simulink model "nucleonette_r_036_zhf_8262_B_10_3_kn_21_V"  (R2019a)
settings: Solver=VariableStepAuto  StartTime=0.0  StopTime=727544.216  FixedStep=0.2  RelTol=1e-6
libraries: simulink x6
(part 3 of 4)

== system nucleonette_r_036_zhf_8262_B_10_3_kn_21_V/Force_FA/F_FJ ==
  In1 : Inport
  Add{12,37,39,52} (4 alike) : Sum
  Add33 : Sum  Inputs=-+
  C_10 : Constant  Value=10
  C_100 : Constant  Value=-100
  C_10_11 : Constant  Value=1E-21
  Clock1 : Clock
  Constant10 : Constant  Value=0.86602
  Constant13 : Constant  Value=3
  Constant15 : Constant  Value=1.0E-3
  Constant19 : Constant  Value=2
  Constant21 : Constant  Value=1.5
  Constant24 : Constant  Value=3
  Math Function25 : Math  Operator=square
  Math Function28 : Math  Operator=square
  Math Function33 : Math  Operator=pow
  Math Function38 : Math  Operator=pow
  Math Function4 : Math  Operator=square
  Math Function45 : Math  Operator=pow
  Nfjx/Dfjx_3 : Scope
  Omega_w1 : Constant  Value=0.00003453723537
  Product25 : Product  Inputs=**/
  Product28 : Product  Inputs=*/
  Product31 : Product  Inputs=/**
  Product{32,53,57,59,61} (5 alike) : Product
  Product44 : Product  Inputs=**/
  Product51 : Product  Inputs=*/*
  Product58 : Product  Inputs=3
  Sqrt11 : Sqrt
  Sqrt13 : Sqrt
  Trigonometric Function10 : Trigonometry  Operator=cos
  ex : Constant  Value=1.602176565
  kFJx : Constant  Value=7.39283526
  mFAx : Constant  Value=999.755388642
  rx1 : Constant  Value=0.36373
  Out1 : Outport
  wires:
  Sqrt11/1 -> Product51/3, Math Function33/1  "Dfj"
  Constant13/1 -> Sqrt13/1, Product32/2
  Constant15/1 -> Math Function45/1
  Product25/1 -> Product32/1  "r*cos(wt)/2"
  Add33/1 -> Math Function25/1
  kFJx/1 -> Product31/3
  Product59/1 -> Add12/1  "3*z/2"
  Add12/1 -> Math Function28/1, Product61/2  "Zfj"
  Product32/1 -> Add33/2  "3r*cos(wt)/2"
  Product61/1 -> Product28/1
  Constant24/1 -> Math Function33/2, Math Function45/2
  Add52/1 -> Product28/2  "Dfj_B"
  C_10_11/1 -> Add39/1
  Add39/1 -> Product53/1  "kn_Dfj"
  Math Function25/1 -> Add37/2
  Math Function28/1 -> Add37/1
  Math Function4/1 -> Product31/2
  Clock1/1 -> Product57/1
  Product58/1 -> Add12/2  "r*cos(wt)*sqrt(3)/2"
  Sqrt13/1 -> Product44/2  "sqrt(3)"
  C_100/1 -> Product51/1
  Product57/1 -> Trigonometric Function10/1  "angle_wt"
  Product44/1 -> Add33/1  "z*sqrt(3)/2"
  Math Function45/1 -> Add52/1
  Math Function33/1 -> Add52/2
  ex/1 -> Math Function4/1
  Constant19/1 -> Product25/3, Product44/3  "2"
  Trigonometric Function10/1 -> Product58/2, Product25/1  "cos(wt)"
  Constant10/1 -> Product58/1  "sqrt(3)/2"
  Product53/1 -> Product61/1
  Product28/1 -> Out1/1, Nfjx/Dfjx_3/1  "nfjx/dfjx_3"
  Omega_w1/1 -> Product57/2
  Add37/1 -> Sqrt11/1
  C_10/1 -> Math Function38/1
  Math Function38/1 -> Add39/2  "10_exp(-100Dfj/r)"
  Product51/1 -> Math Function38/2
  rx1/1 -> Product51/2, Product58/3, Product25/2  "rx"
  mFAx/1 -> Product31/1  "mx"
  Product31/1 -> Product53/2
  In1/1 -> Product59/2, Product44/1
  Constant21/1 -> Product59/1

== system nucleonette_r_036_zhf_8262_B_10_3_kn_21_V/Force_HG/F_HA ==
  In1 : Inport
  In2 : Inport  Port=2
  Add10 : Sum  Inputs=--+
  Add11 : Sum  Inputs=+-+
  Add15 : Sum
  Add19 : Sum
  Add20 : Sum
  Add3 : Sum  Inputs=+++
  Add7 : Sum  Inputs=-+
  C_100 : Constant  Value=-100
  C_10_11_1 : Constant  Value=1E-21
  Clock : Clock
  Constant1 : Constant  Value=10
  Constant15 : Constant  Value=1.0E-3
  Constant16 : Constant  Value=0.86602
  Constant22 : Constant  Value=2
  Constant24 : Constant  Value=3
  Constant5 : Constant  Value=2
  Constant8 : Constant  Value=3
  Constant9 : Constant  Value=3
  Math Function{2,7,9,13} (4 alike) : Math  Operator=square
  Math Function18 : Math  Operator=pow
  Math Function45 : Math  Operator=pow
  Math Function8 : Math  Operator=pow
  Nhax/Dhax_3 : Scope
  Omega_w : Constant  Value=0.00003453723537
  Product{1,16,43,74} (4 alike) : Product  Inputs=**
  Product{5,11,19,30,39} (5 alike) : Product
  Product22 : Product  Inputs=*/
  Product24 : Product  Inputs=*/
  Product35 : Product  Inputs=/**
  Product36 : Product  Inputs=/*
  Product38 : Product  Inputs=***
  Product41 : Product  Inputs=**/
  Product72 : Product  Inputs=*/*
  Sqrt1 : Sqrt
  Sqrt7 : Sqrt
  Subtract7 : Sum
  Trigonometric Function1 : Trigonometry
  Trigonometric Function2 : Trigonometry  Operator=cos
  Trigonometric Function3 : Trigonometry
  Trigonometric Function6 : Trigonometry  Operator=cos
  ex_1 : Constant  Value=1.602176565
  keHAx : Constant  Value=66.535517341
  mHG0 : Constant  Value=707.811386658
  rx : Constant  Value=0.36373
  Out1 : Outport
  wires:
  Product16/1 -> Add19/2  "r*sin(3wt)"
  Omega_w/1 -> Product5/2
  Subtract7/1 -> Product22/2
  Add20/1 -> Add7/2  "z/2 + z0 - z3"
  Math Function8/1 -> Subtract7/1  "Dhax_3"
  Product22/1 -> Nhax/Dhax_3/1, Out1/1  "nhax/dhax_3"
  keHAx/1 -> Product35/3
  Product1/1 -> Add10/1  "(z0-z3)*sqrt(3)/2"
  Trigonometric Function6/1 -> Product38/1, Product43/2  "cos(wt)"
  Add11/1 -> Math Function7/1  "Zha"
  Product43/1 -> Add10/3  "r*cos(wt)"
  Product41/1 -> Add10/2, Product30/1  "r*cos(3wt)/2"
  Product11/1 -> Add19/1  "r*sin(wt)"
  Math Function13/1 -> Product35/2
  Math Function18/1 -> Add15/1  "10_exp(-100Dha/r)"
  Trigonometric Function2/1 -> Product41/1  "cos(3wt)"
  Math Function9/1 -> Add3/2  "Xha_2"
  Product36/1 -> Add20/2  "z/2"
  Product24/1 -> Add11/1, Product1/2  "(z0-z3)/2"
  Constant8/1 -> Sqrt7/1, Product19/2
  Product39/1 -> Product22/1  "Nha"
  ex_1/1 -> Math Function13/1
  Product74/1 -> Product39/1  "kn_Dha"
  Trigonometric Function1/1 -> Product16/2  "sin(3wt)"
  Add3/1 -> Sqrt1/1  "Dhax_2"
  Math Function7/1 -> Add3/3  "Zha_2"
  Constant22/1 -> Product36/1
  Product38/1 -> Add7/1  "r*cos(wt)*sqrt(3)/2"
  Math Function2/1 -> Add3/1
  rx/1 -> Product41/2, Product43/1, Product72/2, Product38/2, Product16/1, Product11/2  "rx"
  Clock/1 -> Product5/1
  Add10/1 -> Math Function9/1  "Xha"
  Product72/1 -> Math Function18/2
  Constant16/1 -> Product38/3  "sqrt(3)/2"
  Trigonometric Function3/1 -> Product11/1  "sin(wt)"
  Product19/1 -> Trigonometric Function2/1, Trigonometric Function1/1
  Constant5/1 -> Product41/3, Product24/2  "2"
  Product35/1 -> Product74/2
  C_10_11_1/1 -> Add15/2
  mHG0/1 -> Product35/1  "mx"
  Add15/1 -> Product74/1
  Sqrt1/1 -> Math Function8/1, Product72/1  "Dhax"
  Sqrt7/1 -> Product30/2, Product1/1  "sqrt(3)"
  Constant9/1 -> Math Function8/2
  Add19/1 -> Math Function2/1  "r*sin(3wt) + r*sin(wt)"
  Product30/1 -> Add11/2  "r*cos(3wt)*sqrt(3)/2"
  Product5/1 -> Trigonometric Function6/1, Trigonometric Function3/1, Product19/1  "ai+wt"
  In2/1 -> Product24/1, Add20/1  "z0 - Z3"
  In1/1 -> Add11/3, Product36/2  "z"
  Add7/1 -> Product39/2
  C_100/1 -> Product72/3
  Constant1/1 -> Math Function18/1
  Constant15/1 -> Math Function45/1
  Constant24/1 -> Math Function45/2
  Math Function45/1 -> Subtract7/2

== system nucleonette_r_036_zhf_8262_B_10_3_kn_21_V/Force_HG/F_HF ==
  In1 : Inport
  In2 : Inport  Port=2
  Add13 : Sum  Inputs=+++
  Add14 : Sum  Inputs=+-+
  Add16 : Sum
  Add20 : Sum
  Add5 : Sum  Inputs=+++
  Add6 : Sum
  Add9 : Sum  Inputs=+-
  C_100 : Constant  Value=-100
  C_10_11_1 : Constant  Value=1E-21
  Clock : Clock
  Constant : Constant  Value=10
  Constant15 : Constant  Value=1.0E-3
  Constant16 : Constant  Value=0.86602
  Constant22 : Constant  Value=2
  Constant24 : Constant  Value=3
  Constant5 : Constant  Value=2
  Constant8 : Constant  Value=3
  Constant9 : Constant  Value=3
  Math Function{10..11,13,15} (4 alike) : Math  Operator=square
  Math Function12 : Math  Operator=pow
  Math Function19 : Math  Operator=pow
  Math Function45 : Math  Operator=pow
  Nhfx/Dhfx_3 : Scope
  Omega_w : Constant  Value=0.00003453723537
  Product{1,16,42..43,73} (5 alike) : Product  Inputs=**
  Product{5,19,30,37} (4 alike) : Product
  Product24 : Product  Inputs=*/
  Product34 : Product  Inputs=*/
  Product35 : Product  Inputs=/**
  Product36 : Product  Inputs=/*
  Product38 : Product  Inputs=***
  Product41 : Product  Inputs=**/
  Product49 : Product  Inputs=**/
  Sqrt7 : Sqrt
  Sqrt8 : Sqrt
  Subtract8 : Sum
  Trigonometric Function1 : Trigonometry
  Trigonometric Function2 : Trigonometry  Operator=cos
  Trigonometric Function5 : Trigonometry
  Trigonometric Function6 : Trigonometry  Operator=cos
  ex_1 : Constant  Value=1.602176565
  keHFx : Constant  Value=66.535517341
  mHG0 : Constant  Value=707.811386658
  rx : Constant  Value=0.36373
  Out1 : Outport
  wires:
  Constant15/1 -> Math Function45/1
  Product16/1 -> Add9/1  "r*sin(3wt)"
  Omega_w/1 -> Product5/2
  Add20/1 -> Add6/2  "z/2 + z0 - z3"
  keHFx/1 -> Product35/3
  Sqrt8/1 -> Product49/1, Math Function12/1  "Dhfx"
  Product1/1 -> Add13/1  "(z0-z3)*sqrt(3)/2"
  Add9/1 -> Math Function10/1  "r*sin(3wt) - r*sin(wt)"
  Trigonometric Function6/1 -> Product38/1, Product43/2  "cos(wt)"
  Add5/1 -> Sqrt8/1  "Dhfx_2"
  Product43/1 -> Add13/2  "r*cos(wt)"
  Product41/1 -> Product30/1, Add13/3  "r*cos(3wt)/2"
  Math Function13/1 -> Product35/2
  Trigonometric Function2/1 -> Product41/1  "cos(3wt)"
  Product36/1 -> Add20/2  "z/2"
  Product24/1 -> Add14/1, Product1/2  "(z0-z3)/2"
  Constant8/1 -> Sqrt7/1, Product19/2
  Product34/1 -> Out1/1, Nhfx/Dhfx_3/1  "Nhfx/Dhfx_3"
  ex_1/1 -> Math Function13/1
  Product5/1 -> Trigonometric Function6/1, Product19/1, Trigonometric Function5/1  "ai+wt"
  Product42/1 -> Add9/2  "r*sin(wt)"
  Trigonometric Function1/1 -> Product16/2  "sin(3wt)"
  Product73/1 -> Product37/1  "kn_Dhf"
  Trigonometric Function5/1 -> Product42/1  "sin(wt)"
  Math Function11/1 -> Add5/2  "Xhf_2"
  Add13/1 -> Math Function11/1  "Xhf"
  Constant22/1 -> Product36/1
  Product38/1 -> Add6/1  "r*cos(wt)*sqrt(3)/2"
  Constant24/1 -> Math Function45/2
  rx/1 -> Product38/2, Product49/3, Product42/2, Product43/1, Product16/1, Product41/2  "rx"
  Add16/1 -> Product73/1
  Clock/1 -> Product5/1
  Product37/1 -> Product34/1  "Nhf"
  Constant16/1 -> Product38/3  "sqrt(3)/2"
  Product19/1 -> Trigonometric Function2/1, Trigonometric Function1/1
  Constant5/1 -> Product24/2, Product41/3  "2"
  In2/1 -> Add20/1, Product24/1  "z0 - z3"
  Product35/1 -> Product73/2
  C_10_11_1/1 -> Add16/2
  mHG0/1 -> Product35/1  "mx"
  Add6/1 -> Product37/2
  Add14/1 -> Math Function15/1  "Zhf"
  Product49/1 -> Math Function19/2
  Math Function19/1 -> Add16/1  "10_exp(-100Dhf/r)"
  Sqrt7/1 -> Product30/2, Product1/1  "sqrt(3)"
  Math Function15/1 -> Add5/3  "Zhf_2"
  Constant9/1 -> Math Function12/2
  Product30/1 -> Add14/2  "r*cos(3wt)*sqrt(3)/2"
  Math Function10/1 -> Add5/1  "Yhf_2"
  Math Function45/1 -> Subtract8/2
  Math Function12/1 -> Subtract8/1  "Dhfx_3"
  Subtract8/1 -> Product34/2
  In1/1 -> Add14/3, Product36/2
  C_100/1 -> Product49/2
  Constant/1 -> Math Function19/1

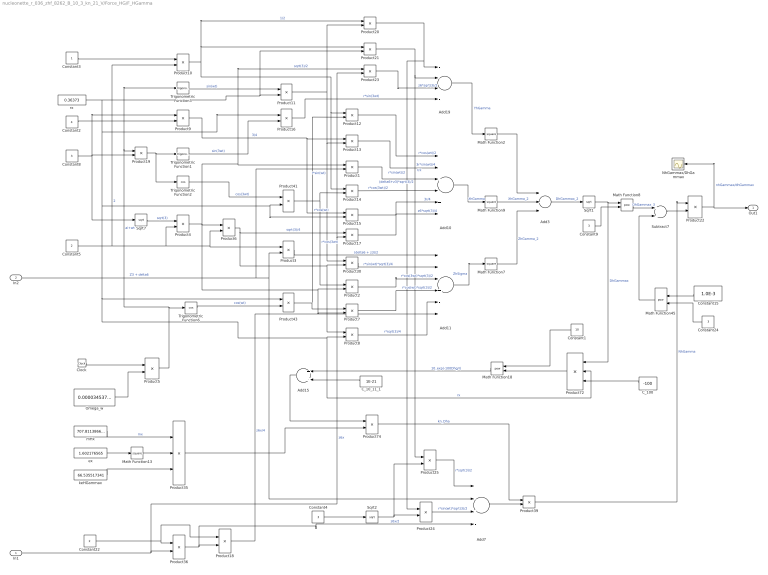
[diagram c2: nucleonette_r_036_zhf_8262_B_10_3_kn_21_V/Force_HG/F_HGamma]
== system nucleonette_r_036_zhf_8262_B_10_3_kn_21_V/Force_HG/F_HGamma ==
  In1 : Inport
  In2 : Inport  Port=2
  Add10 : Sum  Inputs=+-+-++
  Add11 : Sum  Inputs=-+-+--
  Add15 : Sum
  Add19 : Sum  Inputs=----
  Add3 : Sum  Inputs=+++
  Add7 : Sum  Inputs=--+-
  C_100 : Constant  Value=-100
  C_10_11_1 : Constant  Value=1E-21
  Clock : Clock
  Constant1 : Constant  Value=10
  Constant15 : Constant  Value=1.0E-3
  Constant2 : Constant  Value=4
  Constant22 : Constant  Value=2
  Constant{4,8..9,24} (4 alike) : Constant  Value=3
  Constant3 : Constant
  Constant5 : Constant  Value=2
  Math Function{2,7,9,13} (4 alike) : Math  Operator=square
  Math Function18 : Math  Operator=pow
  Math Function45 : Math  Operator=pow
  Math Function8 : Math  Operator=pow
  NhGammax/DhGammax : Scope
  Omega_w : Constant  Value=0.00003453723537
  Product{1,12..17,20..21,23..25,41,43,74} (15 alike) : Product  Inputs=**
  Product{4,6,9..10,22} (5 alike) : Product  Inputs=*/
  Product{2,5,7..8,11,19,30,39} (8 alike) : Product
  Product18 : Product  Inputs=/*
  Product3 : Product  Inputs=/*
  Product35 : Product  Inputs=/**
  Product36 : Product  Inputs=/*
  Product72 : Product  Inputs=*/*
  Sqrt1 : Sqrt
  Sqrt2 : Sqrt
  Sqrt7 : Sqrt
  Subtract7 : Sum
  Trigonometric Function1 : Trigonometry
  Trigonometric Function2 : Trigonometry  Operator=cos
  Trigonometric Function3 : Trigonometry
  Trigonometric Function6 : Trigonometry  Operator=cos
  ex : Constant  Value=1.602176565
  keHGammax : Constant  Value=66.535517341
  mHx : Constant  Value=707.811386658
  rx : Constant  Value=0.36373
  Out1 : Outport
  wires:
  Product15/1 -> Add10/5  "3r/4"
  Product18/1 -> Add11/6  "z6x/4"
  Constant4/1 -> Sqrt2/1
  Product4/1 -> Product7/2, Product2/2, Product6/1, Product23/1, Product1/1  "sqrt(3)/2"
  Product36/1 -> Add7/4, Product18/2  "z6x/2"
  Product3/1 -> Add11/1  "(delta6 + z3)/2"
  Constant2/1 -> Product9/2
  Product21/1 -> Add19/2, Product25/1  "r/2"
  Product23/1 -> Add19/3  "z6*sqrt(3)/2"
  Product16/1 -> Add19/4  "r*sin(3wt)"
  Product10/1 -> Product14/1, Product12/1, Product20/1, Product21/1  "1/2"
  Product13/1 -> Add10/2  "3r*sin(wt)/4"
  Product20/1 -> Add19/1, Product24/1  "r*sin(wt)/2"
  Sqrt2/1 -> Product25/2, Product24/2
  Product12/1 -> Add10/1  "r*cos(wt)/2"
  Product8/1 -> Add11/5  "r*sqrt(3)/4"
  Product7/1 -> Add11/4  "r*cos(wt)*sqrt(3)/2"
  Product9/1 -> Product15/1, Product13/1  "3/4"
  Product2/1 -> Add11/3  "r*cos(3wt)*sqrt(3)/2"
  Product6/1 -> Product17/1, Product8/1, Product30/2  "sqrt(3)/4"
  Product25/1 -> Add7/1  "r*sqrt(3)/2"
  Math Function45/1 -> Subtract7/2
  Constant24/1 -> Math Function45/2
  Constant1/1 -> Math Function18/1
  Constant15/1 -> Math Function45/1
  ex/1 -> Math Function13/1
  Add7/1 -> Product39/2
  C_10_11_1/1 -> Add15/2
  Add19/1 -> Math Function2/1  "YhGamma"
  Constant3/1 -> Product10/1
  Constant8/1 -> Product9/1, Sqrt7/1, Product19/2
  In1/1 -> Product17/2, Product23/2, Product36/2  "z6x"
  Product24/1 -> Add7/3  "r*sin(wt)*sqrt(3)/2"
  In2/1 -> Product1/2, Add7/2, Product3/2  "Z3 + delta6"
  Math Function7/1 -> Add3/3  "ZhGamma_2"
  Product19/1 -> Trigonometric Function2/1, Trigonometric Function1/1
  Subtract7/1 -> Product22/2
  Constant9/1 -> Math Function8/2
  Add15/1 -> Product74/1
  Product22/1 -> NhGammax/DhGammax/1, Out1/1  "nhGammax/dhGammax"
  Sqrt7/1 -> Product4/1  "sqrt(3)"
  Product35/1 -> Product74/2
  Product1/1 -> Add10/3  "(delta6+z3)*sqrt(3)/2"
  Constant5/1 -> Product10/2, Product4/2, Product3/1, Product6/2  "2"
  Trigonometric Function3/1 -> Product11/1  "sin(wt)"
  Product5/1 -> Trigonometric Function6/1, Trigonometric Function3/1, Product19/1  "ai+wt"
  Product30/1 -> Add11/2  "r*sin(wt)*sqrt(3)/4"
  Product43/1 -> Product12/2, Product7/1  "r*cos(wt)"
  Product41/1 -> Product14/2, Product2/1  "r*cos(3wt)"
  Product72/1 -> Math Function18/2
  Add10/1 -> Math Function9/1  "XhGamma"
  Clock/1 -> Product5/1
  rx/1 -> Product43/1, Product8/2, Product72/2, Product15/2, Product41/2, Product16/1, Product21/2, Product11/2  "rx"
  Trigonometric Function6/1 -> Product43/2  "cos(wt)"
  Math Function2/1 -> Add3/1
  Constant22/1 -> Product18/1, Product36/1
  Math Function18/1 -> Add15/1  "10_exp(-100Dhg/r)"
  Sqrt1/1 -> Math Function8/1, Product72/1  "DhGammax"
  Trigonometric Function1/1 -> Product16/2  "sin(3wt)"
  Add3/1 -> Sqrt1/1  "DhGammax_2"
  Product17/1 -> Add10/6  "z6*sqrt(3)/4"
  Product74/1 -> Product39/1  "kn_Dha"
  C_100/1 -> Product72/3
  Product39/1 -> Product22/1  "NhGamma"
  Add11/1 -> Math Function7/1  "ZhSigma"
  Trigonometric Function2/1 -> Product41/1  "cos(3wt)"
  Math Function9/1 -> Add3/2  "XhGamma_2"
  keHGammax/1 -> Product35/3
  Product11/1 -> Product13/2, Product30/1, Product20/2  "r*sin(wt)"
  Math Function8/1 -> Subtract7/1  "DhGammax_3"
  Math Function13/1 -> Product35/2
  Product14/1 -> Add10/4  "r*cos(3wt)/2"
  mHx/1 -> Product35/1  "mx"
  Omega_w/1 -> Product5/2

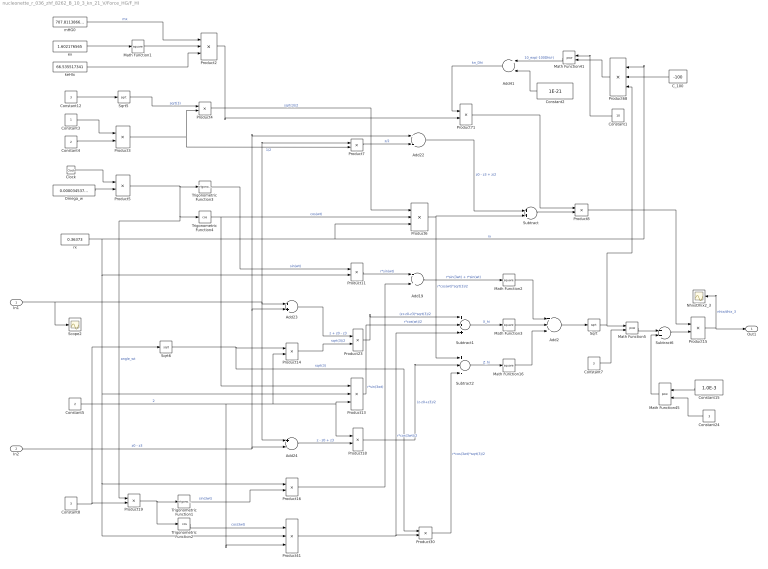
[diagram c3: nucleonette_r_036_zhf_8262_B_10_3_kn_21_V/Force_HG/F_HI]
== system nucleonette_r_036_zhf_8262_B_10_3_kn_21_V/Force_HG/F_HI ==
  In1 : Inport
  In2 : Inport  Port=2
  Add{19,22..23,41} (4 alike) : Sum
  Add2 : Sum  Inputs=+++
  Add24 : Sum  Inputs=+-
  C_100 : Constant  Value=-100
  Clock : Clock
  Constant1 : Constant  Value=10
  Constant{7..8,12,24} (4 alike) : Constant  Value=3
  Constant15 : Constant  Value=1.0E-3
  Constant2 : Constant  Value=1E-21
  Constant3 : Constant
  Constant4 : Constant  Value=2
  Constant5 : Constant  Value=2
  Math Function{1..3,16} (4 alike) : Math  Operator=square
  Math Function41 : Math  Operator=pow
  Math Function45 : Math  Operator=pow
  Math Function5 : Math  Operator=pow
  Nhix/Dhix2_3 : Scope
  Omega_w : Constant  Value=0.00003453723537
  Product{4..5,7..8,11,19,30,71} (8 alike) : Product
  Product13 : Product  Inputs=**/
  Product14 : Product  Inputs=*/
  Product15 : Product  Inputs=*/
  Product16 : Product  Inputs=**
  Product18 : Product  Inputs=/*
  Product2 : Product  Inputs=/**
  Product23 : Product  Inputs=**
  Product3 : Product  Inputs=*/
  Product41 : Product  Inputs=**/
  Product6 : Product  Inputs=3
  Product68 : Product  Inputs=/**
  Scope2 : Scope
  Sqrt : Sqrt
  Sqrt5 : Sqrt
  Sqrt6 : Sqrt
  Subtract : Sum
  Subtract1 : Sum  Inputs=+++
  Subtract2 : Sum  Inputs=+--
  Subtract6 : Sum
  Trigonometric Function1 : Trigonometry
  Trigonometric Function2 : Trigonometry  Operator=cos
  Trigonometric Function3 : Trigonometry
  Trigonometric Function4 : Trigonometry  Operator=cos
  ex : Constant  Value=1.602176565
  keHIx : Constant  Value=66.535517341
  mHG0 : Constant  Value=707.811386658
  rx : Constant  Value=0.36373
  Out1 : Outport
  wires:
  Sqrt5/1 -> Product4/1  "sqrt(3)"
  Product3/1 -> Product4/2, Product7/2  "1/2"
  Constant15/1 -> Math Function45/1
  Sqrt6/1 -> Product30/1, Product14/1  "sqrt(3)"
  Product41/1 -> Product30/2, Subtract1/3  "r*cos(3wt)/2"
  Subtract/1 -> Product8/2
  Subtract2/1 -> Math Function16/1  "Z_hi"
  Trigonometric Function3/1 -> Product11/1  "sin(wt)"
  Constant7/1 -> Math Function5/2
  Product8/1 -> Product15/1
  Constant24/1 -> Math Function45/2
  Constant4/1 -> Product3/2
  Product13/1 -> Subtract1/2  "r*cos(wt)/2"
  Product2/1 -> Product71/2
  Product6/1 -> Subtract/2, Subtract2/1  "r*cos(wt)*sqrt(3)/2"
  Add41/1 -> Product71/1  "kn_Dhi"
  Product11/1 -> Add19/1  "r*sin(wt)"
  Subtract6/1 -> Product15/2
  Add24/1 -> Product18/2  "z - z0 + z3"
  Math Function41/1 -> Add41/1  "10_exp(-100Dhi/r)"
  Product18/1 -> Subtract2/2  "(z-z0+z3)/2"
  Product14/1 -> Product23/2  "sqrt(3)/2"
  Constant8/1 -> Sqrt6/1, Product19/2
  Product71/1 -> Product8/1
  Add2/1 -> Sqrt/1
  Product4/1 -> Product6/1  "sqrt(3)/2"
  Product23/1 -> Subtract1/1  "(z+z0-z3)*sqrt(3)/2"
  mHG0/1 -> Product2/1  "mx"
  Add22/1 -> Subtract/1  "z0 - z3 + z/2"
  Add19/1 -> Math Function2/1  "r*sin(3wt) + r*sin(wt)"
  Subtract1/1 -> Math Function3/1  "X_hi"
  Omega_w/1 -> Product5/2
  Product19/1 -> Trigonometric Function2/1, Trigonometric Function1/1
  Add23/1 -> Product23/1  "z + z0 - z3"
  keHIx/1 -> Product2/3
  Sqrt/1 -> Math Function5/1, Product68/3
  ex/1 -> Math Function1/1
  Math Function45/1 -> Subtract6/2
  Math Function1/1 -> Product2/2
  Product68/1 -> Math Function41/2
  Math Function16/1 -> Add2/3
  Constant3/1 -> Product3/1
  Trigonometric Function1/1 -> Product16/2  "sin(3wt)"
  Math Function5/1 -> Subtract6/1
  Constant12/1 -> Sqrt5/1
  Product16/1 -> Add19/2  "r*sin(3wt)"
  rx/1 -> Product6/3, Product68/1, Product13/2, Product41/2, Product16/1, Product11/2  "rx"
  Math Function3/1 -> Add2/2
  Product5/1 -> Product19/1, Trigonometric Function4/1, Trigonometric Function3/1  "angle_wt"
  Product15/1 -> Out1/1, Nhix/Dhix2_3/1  "nhix/dhix_3"
  Product30/1 -> Subtract2/3  "r*cos(3wt)*sqrt(3)/2"
  Math Function2/1 -> Add2/1
  Product7/1 -> Add22/2  "z/2"
  Trigonometric Function4/1 -> Product13/1, Product6/2  "cos(wt)"
  C_100/1 -> Product68/2
  Constant5/1 -> Product41/3, Product14/2, Product18/1, Product13/3  "2"
  Clock/1 -> Product5/1
  Trigonometric Function2/1 -> Product41/1  "cos(3wt)"
  In1/1 -> Scope2/1, Product7/1, Add24/1, Add23/1
  In2/1 -> Add22/1, Add23/2, Add24/2  "z0 - z3"
  Constant1/1 -> Math Function41/1
  Constant2/1 -> Add41/2

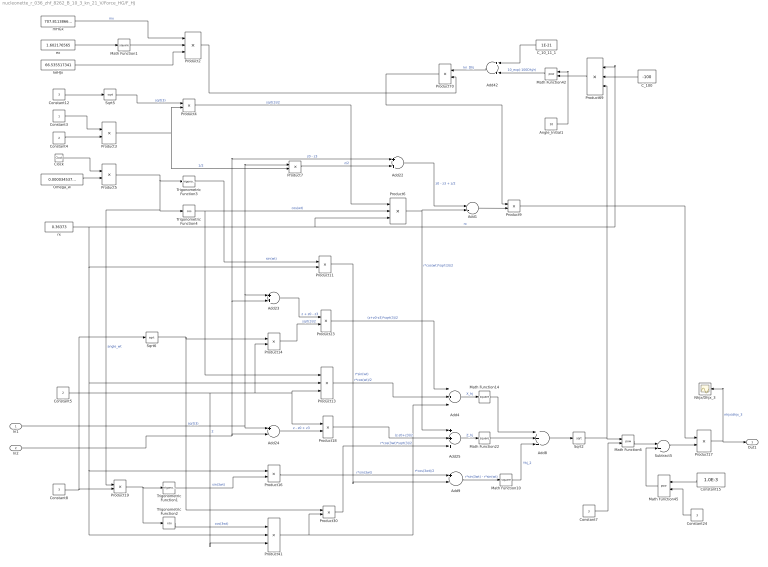
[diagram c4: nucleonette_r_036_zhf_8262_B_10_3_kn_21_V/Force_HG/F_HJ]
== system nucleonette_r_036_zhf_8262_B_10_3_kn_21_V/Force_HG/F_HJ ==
  In1 : Inport
  In2 : Inport  Port=2
  Add1 : Sum  Inputs=+-
  Add22 : Sum
  Add23 : Sum
  Add24 : Sum  Inputs=+-
  Add25 : Sum  Inputs=+++
  Add4 : Sum  Inputs=-+-
  Add42 : Sum
  Add8 : Sum  Inputs=+++
  Add9 : Sum  Inputs=+-
  Angle_Initial1 : Constant  Value=10
  C_100 : Constant  Value=-100
  C_10_11_1 : Constant  Value=1E-21
  Clock : Clock
  Constant{7..8,12,24} (4 alike) : Constant  Value=3
  Constant15 : Constant  Value=1.0E-3
  Constant3 : Constant
  Constant4 : Constant  Value=2
  Constant5 : Constant  Value=2
  Math Function{1,10,14,22} (4 alike) : Math  Operator=square
  Math Function42 : Math  Operator=pow
  Math Function45 : Math  Operator=pow
  Math Function6 : Math  Operator=pow
  Nhjx/Dhjx_3 : Scope
  Omega_w : Constant  Value=0.00003453723537
  Product{4..5,7,9,11,19,30,70} (8 alike) : Product
  Product13 : Product  Inputs=**/
  Product14 : Product  Inputs=*/
  Product16 : Product  Inputs=**
  Product17 : Product  Inputs=*/
  Product18 : Product  Inputs=/*
  Product2 : Product  Inputs=/**
  Product23 : Product  Inputs=**
  Product3 : Product  Inputs=*/
  Product41 : Product  Inputs=**/
  Product6 : Product  Inputs=3
  Product69 : Product  Inputs=/**
  Sqrt2 : Sqrt
  Sqrt5 : Sqrt
  Sqrt6 : Sqrt
  Subtract5 : Sum
  Trigonometric Function1 : Trigonometry
  Trigonometric Function2 : Trigonometry  Operator=cos
  Trigonometric Function3 : Trigonometry
  Trigonometric Function4 : Trigonometry  Operator=cos
  ex : Constant  Value=1.602176565
  keHJx : Constant  Value=66.535517341
  mHGx : Constant  Value=707.811386658
  rx : Constant  Value=0.36373
  Out1 : Outport
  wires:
  Product70/1 -> Product9/1
  Sqrt2/1 -> Product69/3, Math Function6/1
  Sqrt5/1 -> Product4/1  "sqrt(3)"
  Product3/1 -> Product4/2, Product7/2  "1/2"
  Constant15/1 -> Math Function45/1
  Sqrt6/1 -> Product14/1, Product30/1  "sqrt(3)"
  Product41/1 -> Product30/2, Add4/3  "r*cos(3wt)/2"
  Trigonometric Function3/1 -> Product11/1  "sin(wt)"
  Constant7/1 -> Math Function6/2
  Constant24/1 -> Math Function45/2
  Constant4/1 -> Product3/2
  Product13/1 -> Add4/2  "r*cos(wt)/2"
  Product2/1 -> Product70/2
  Product6/1 -> Add25/1, Add1/2  "r*cos(wt)*sqrt(3)/2"
  Product11/1 -> Add9/2  "r*sin(wt)"
  Add24/1 -> Product18/2  "z - z0 + z3"
  Product18/1 -> Add25/2  "(z-z0+z3)/2"
  Product14/1 -> Product23/2  "sqrt(3)/2"
  Math Function14/1 -> Add8/1
  Constant8/1 -> Sqrt6/1, Product19/2
  Add4/1 -> Math Function14/1  "X_hj"
  Product4/1 -> Product6/1  "sqrt(3)/2"
  Product23/1 -> Add4/1  "(z+z0-z3)*sqrt(3)/2"
  mHGx/1 -> Product2/1  "mx"
  Add22/1 -> Add1/1  "z0 - z3 + z/2"
  Product69/1 -> Math Function42/2
  Subtract5/1 -> Product17/2
  Omega_w/1 -> Product5/2
  Math Function22/1 -> Add8/2
  Product19/1 -> Trigonometric Function2/1, Trigonometric Function1/1
  Add23/1 -> Product23/1  "z + z0 - z3"
  Add42/1 -> Product70/1  "kn_Dhj"
  keHJx/1 -> Product2/3
  Add25/1 -> Math Function22/1  "Z_hj"
  Math Function42/1 -> Add42/2  "10_exp(-100Dhj/r)"
  ex/1 -> Math Function1/1
  Math Function45/1 -> Subtract5/2
  Math Function6/1 -> Subtract5/1
  Math Function1/1 -> Product2/2
  Product17/1 -> Out1/1, Nhjx/Dhjx_3/1  "nhjx/dhjx_3"
  Add8/1 -> Sqrt2/1
  Constant3/1 -> Product3/1
  Trigonometric Function1/1 -> Product16/2  "sin(3wt)"
  Constant12/1 -> Sqrt5/1
  Product16/1 -> Add9/1  "r*sin(3wt)"
  Add1/1 -> Product9/2
  rx/1 -> Product13/2, Product41/2, Product16/1, Product11/2, Product6/3, Product69/1  "rx"
  Add9/1 -> Math Function10/1  "r*sin(3wt) - r*sin(wt)"
  Product5/1 -> Trigonometric Function3/1, Trigonometric Function4/1, Product19/1  "angle_wt"
  Product30/1 -> Add25/3  "r*cos(3wt)*sqrt(3)/2"
  Product7/1 -> Add22/2  "z/2"
  Trigonometric Function4/1 -> Product13/1, Product6/2  "cos(wt)"
  C_100/1 -> Product69/2
  Product9/1 -> Product17/1
  Constant5/1 -> Product41/3, Product14/2, Product13/3, Product18/1  "2"
  Math Function10/1 -> Add8/3  "Yhj_2"
  Clock/1 -> Product5/1
  Trigonometric Function2/1 -> Product41/1  "cos(3wt)"
  C_10_11_1/1 -> Add42/1
  In1/1 -> Product7/1, Add23/1, Add24/1
  In2/1 -> Add22/1, Add23/2, Add24/2  "z0 - z3"
  Angle_Initial1/1 -> Math Function42/1

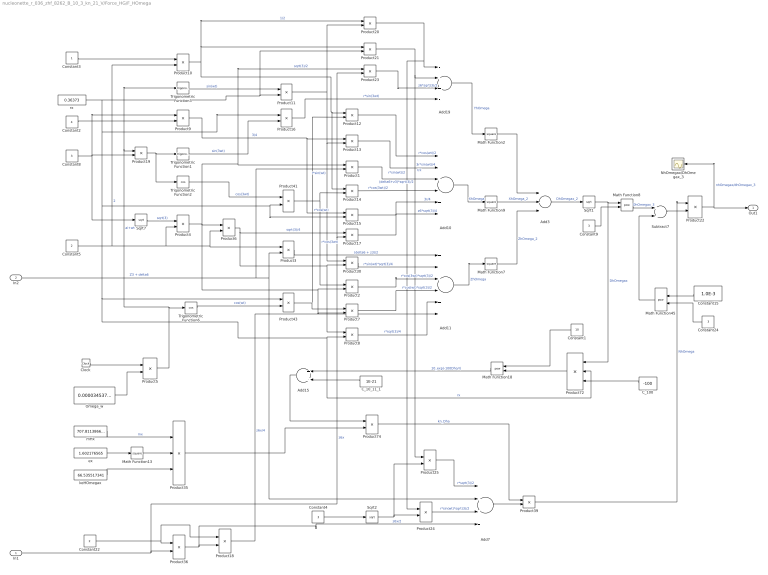
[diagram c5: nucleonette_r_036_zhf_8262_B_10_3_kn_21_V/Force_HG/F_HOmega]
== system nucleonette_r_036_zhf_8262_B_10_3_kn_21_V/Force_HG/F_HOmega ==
  In1 : Inport
  In2 : Inport  Port=2
  Add10 : Sum  Inputs=+++-++
  Add11 : Sum  Inputs=+++-++
  Add15 : Sum
  Add19 : Sum  Inputs=-++-
  Add3 : Sum  Inputs=+++
  Add7 : Sum  Inputs=++++
  C_100 : Constant  Value=-100
  C_10_11_1 : Constant  Value=1E-21
  Clock : Clock
  Constant1 : Constant  Value=10
  Constant15 : Constant  Value=1.0E-3
  Constant2 : Constant  Value=4
  Constant22 : Constant  Value=2
  Constant{4,8..9,24} (4 alike) : Constant  Value=3
  Constant3 : Constant
  Constant5 : Constant  Value=2
  Math Function{2,7,9,13} (4 alike) : Math  Operator=square
  Math Function18 : Math  Operator=pow
  Math Function45 : Math  Operator=pow
  Math Function8 : Math  Operator=pow
  NhOmegax/DhOmegax_3 : Scope
  Omega_w : Constant  Value=0.00003453723537
  Product{1,12..17,20..21,23..25,41,43,74} (15 alike) : Product  Inputs=**
  Product{4,6,9..10,22} (5 alike) : Product  Inputs=*/
  Product{2,5,7..8,11,19,30,39} (8 alike) : Product
  Product18 : Product  Inputs=/*
  Product3 : Product  Inputs=/*
  Product35 : Product  Inputs=/**
  Product36 : Product  Inputs=/*
  Product72 : Product  Inputs=*/*
  Sqrt1 : Sqrt
  Sqrt2 : Sqrt
  Sqrt7 : Sqrt
  Subtract7 : Sum
  Trigonometric Function1 : Trigonometry
  Trigonometric Function2 : Trigonometry  Operator=cos
  Trigonometric Function3 : Trigonometry
  Trigonometric Function6 : Trigonometry  Operator=cos
  ex : Constant  Value=1.602176565
  keHOmegax : Constant  Value=66.535517341
  mHx : Constant  Value=707.811386658
  rx : Constant  Value=0.36373
  Out1 : Outport
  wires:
  Product15/1 -> Add10/5  "3r/4"
  Product18/1 -> Add11/6  "z6x/4"
  Constant4/1 -> Sqrt2/1
  Product4/1 -> Product7/2, Product2/2, Product6/1, Product23/1, Product1/1  "sqrt(3)/2"
  Product36/1 -> Add7/4, Product18/2  "z6x/2"
  Product3/1 -> Add11/1  "(delta6 + z3)/2"
  Constant2/1 -> Product9/2
  Product21/1 -> Add19/2, Product25/1  "r/2"
  Product23/1 -> Add19/3  "z6*sqrt(3)/2"
  Product16/1 -> Add19/4  "r*sin(3wt)"
  Product10/1 -> Product14/1, Product12/1, Product20/1, Product21/1  "1/2"
  Product13/1 -> Add10/2  "3r*sin(wt)/4"
  Product20/1 -> Add19/1, Product24/1  "r*sin(wt)/2"
  Sqrt2/1 -> Product25/2, Product24/2
  Product12/1 -> Add10/1  "r*cos(wt)/2"
  Product8/1 -> Add11/5  "r*sqrt(3)/4"
  Product7/1 -> Add11/4  "r*cos(wt)*sqrt(3)/2"
  Product9/1 -> Product15/1, Product13/1  "3/4"
  Product2/1 -> Add11/3  "r*cos(3wt)*sqrt(3)/2"
  Product6/1 -> Product17/1, Product8/1, Product30/2  "sqrt(3)/4"
  Product25/1 -> Add7/1  "r*sqrt(3)/2"
  Math Function45/1 -> Subtract7/2
  Constant24/1 -> Math Function45/2
  Constant1/1 -> Math Function18/1
  Constant15/1 -> Math Function45/1
  ex/1 -> Math Function13/1
  Add7/1 -> Product39/2
  C_10_11_1/1 -> Add15/2
  Add19/1 -> Math Function2/1  "YhOmega"
  Constant3/1 -> Product10/1
  Constant8/1 -> Product9/1, Sqrt7/1, Product19/2
  In1/1 -> Product17/2, Product23/2, Product36/2  "z6x"
  Product24/1 -> Add7/3  "r*sin(wt)*sqrt(3)/2"
  In2/1 -> Product1/2, Add7/2, Product3/2  "Z3 + delta6"
  Math Function7/1 -> Add3/3  "ZhOmega_2"
  Product19/1 -> Trigonometric Function2/1, Trigonometric Function1/1
  Subtract7/1 -> Product22/2
  Constant9/1 -> Math Function8/2
  Add15/1 -> Product74/1
  Product22/1 -> NhOmegax/DhOmegax_3/1, Out1/1  "nhOmegax/dhOmegax_3"
  Sqrt7/1 -> Product4/1  "sqrt(3)"
  Product35/1 -> Product74/2
  Product1/1 -> Add10/3  "(delta6+z3)*sqrt(3)/2"
  Constant5/1 -> Product10/2, Product4/2, Product3/1, Product6/2  "2"
  Trigonometric Function3/1 -> Product11/1  "sin(wt)"
  Product5/1 -> Trigonometric Function6/1, Trigonometric Function3/1, Product19/1  "ai+wt"
  Product30/1 -> Add11/2  "r*sin(wt)*sqrt(3)/4"
  Product43/1 -> Product12/2, Product7/1  "r*cos(wt)"
  Product41/1 -> Product14/2, Product2/1  "r*cos(3wt)"
  Product72/1 -> Math Function18/2
  Add10/1 -> Math Function9/1  "XhOmega"
  Clock/1 -> Product5/1
  rx/1 -> Product43/1, Product8/2, Product72/2, Product15/2, Product41/2, Product16/1, Product21/2, Product11/2  "rx"
  Trigonometric Function6/1 -> Product43/2  "cos(wt)"
  Math Function2/1 -> Add3/1
  Constant22/1 -> Product18/1, Product36/1
  Math Function18/1 -> Add15/1  "10_exp(-100Dho/r)"
  Sqrt1/1 -> Math Function8/1, Product72/1  "DhOmegax"
  Trigonometric Function1/1 -> Product16/2  "sin(3wt)"
  Add3/1 -> Sqrt1/1  "DhOmegax_2"
  Product17/1 -> Add10/6  "z6*sqrt(3)/4"
  Product74/1 -> Product39/1  "kn_Dha"
  C_100/1 -> Product72/3
  Product39/1 -> Product22/1  "NhOmega"
  Add11/1 -> Math Function7/1  "ZhOmega"
  Trigonometric Function2/1 -> Product41/1  "cos(3wt)"
  Math Function9/1 -> Add3/2  "XhOmega_2"
  keHOmegax/1 -> Product35/3
  Product11/1 -> Product13/2, Product30/1, Product20/2  "r*sin(wt)"
  Math Function8/1 -> Subtract7/1  "DhOmegax_3"
  Math Function13/1 -> Product35/2
  Product14/1 -> Add10/4  "r*cos(3wt)/2"
  mHx/1 -> Product35/1  "mx"
  Omega_w/1 -> Product5/2

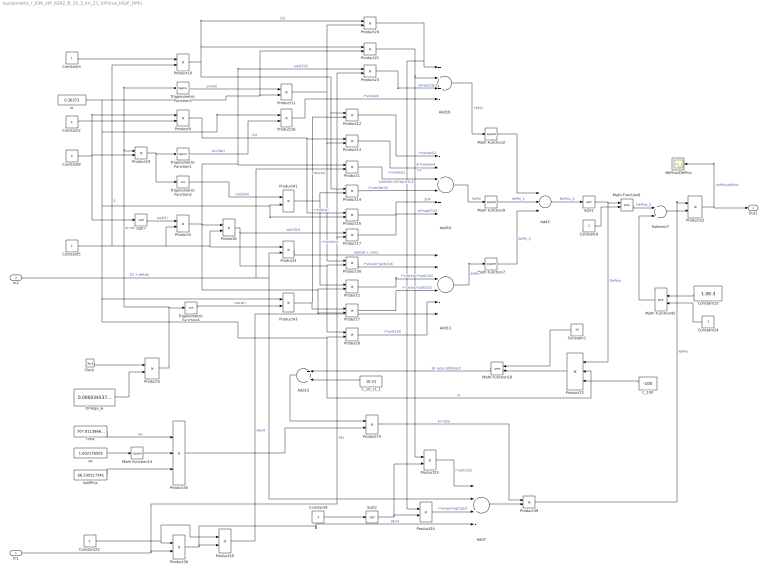
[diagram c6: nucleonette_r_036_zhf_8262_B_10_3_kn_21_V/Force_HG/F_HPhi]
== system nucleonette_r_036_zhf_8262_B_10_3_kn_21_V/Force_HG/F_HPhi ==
  In1 : Inport
  In2 : Inport  Port=2
  Add10 : Sum  Inputs=--+-++
  Add11 : Sum  Inputs=-+----
  Add15 : Sum
  Add19 : Sum  Inputs=+++-
  Add3 : Sum  Inputs=+++
  Add7 : Sum  Inputs=--+-
  C_100 : Constant  Value=-100
  C_10_11_1 : Constant  Value=1E-21
  Clock : Clock
  Constant1 : Constant  Value=10
  Constant15 : Constant  Value=1.0E-3
  Constant2 : Constant  Value=4
  Constant22 : Constant  Value=2
  Constant{4,8..9,24} (4 alike) : Constant  Value=3
  Constant3 : Constant
  Constant5 : Constant  Value=2
  Math Function{2,7,9,13} (4 alike) : Math  Operator=square
  Math Function18 : Math  Operator=pow
  Math Function45 : Math  Operator=pow
  Math Function8 : Math  Operator=pow
  NhPhix/DhPhix : Scope
  Omega_w : Constant  Value=0.00003453723537
  Product{1,12..17,20..21,23..25,41,43,74} (15 alike) : Product  Inputs=**
  Product{4,6,9..10,22} (5 alike) : Product  Inputs=*/
  Product{2,5,7..8,11,19,30,39} (8 alike) : Product
  Product18 : Product  Inputs=/*
  Product3 : Product  Inputs=/*
  Product35 : Product  Inputs=/**
  Product36 : Product  Inputs=/*
  Product72 : Product  Inputs=*/*
  Sqrt1 : Sqrt
  Sqrt2 : Sqrt
  Sqrt7 : Sqrt
  Subtract7 : Sum
  Trigonometric Function1 : Trigonometry
  Trigonometric Function2 : Trigonometry  Operator=cos
  Trigonometric Function3 : Trigonometry
  Trigonometric Function6 : Trigonometry  Operator=cos
  ex : Constant  Value=1.602176565
  keHPhix : Constant  Value=66.535517341
  mHx : Constant  Value=707.811386658
  rx : Constant  Value=0.36373
  Out1 : Outport
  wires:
  Omega_w/1 -> Product5/2
  mHx/1 -> Product35/1  "mx"
  Product14/1 -> Add10/4  "r*cos(3wt)/2"
  Math Function13/1 -> Product35/2
  Math Function8/1 -> Subtract7/1  "DhPhix_3"
  Product11/1 -> Product13/2, Product30/1, Product20/2  "r*sin(wt)"
  keHPhix/1 -> Product35/3
  Math Function9/1 -> Add3/2  "XhPhi_2"
  Trigonometric Function2/1 -> Product41/1  "cos(3wt)"
  Add11/1 -> Math Function7/1  "ZhPhi"
  Product39/1 -> Product22/1  "NhPhi"
  C_100/1 -> Product72/3
  Product17/1 -> Add10/6  "z6*sqrt(3)/4"
  Product20/1 -> Add19/1, Product24/1  "r*sin(wt)/2"
  Constant24/1 -> Math Function45/2
  Product13/1 -> Add10/2  "3r*sin(wt)/4"
  Sqrt2/1 -> Product25/2, Product24/2
  Product10/1 -> Product14/1, Product12/1, Product20/1, Product21/1  "1/2"
  Add7/1 -> Product39/2
  ex/1 -> Math Function13/1
  Product25/1 -> Add7/1  "r*sqrt(3)/2"
  Product16/1 -> Add19/4  "r*sin(3wt)"
  Product2/1 -> Add11/3  "r*cos(3wt)*sqrt(3)/2"
  Product21/1 -> Add19/2, Product25/1  "r/2"
  Product23/1 -> Add19/3  "z6*sqrt(3)/2"
  Product7/1 -> Add11/4  "r*cos(wt)*sqrt(3)/2"
  Product12/1 -> Add10/1  "r*cos(wt)/2"
  Constant15/1 -> Math Function45/1
  Math Function45/1 -> Subtract7/2
  Product6/1 -> Product17/1, Product8/1, Product30/2  "sqrt(3)/4"
  Product36/1 -> Add7/4, Product18/2  "z6x/2"
  C_10_11_1/1 -> Add15/2
  Product4/1 -> Product7/2, Product2/2, Product6/1, Product23/1, Product1/1  "sqrt(3)/2"
  Product74/1 -> Product39/1  "kn_Dha"
  Constant4/1 -> Sqrt2/1
  Product9/1 -> Product15/1, Product13/1  "3/4"
  Product18/1 -> Add11/6  "z6x/4"
  Product15/1 -> Add10/5  "3r/4"
  Product3/1 -> Add11/1  "(delta6 + z3)/2"
  Add19/1 -> Math Function2/1  "YhPhi"
  Subtract7/1 -> Product22/2
  Sqrt1/1 -> Math Function8/1, Product72/1  "DhPhix"
  Constant3/1 -> Product10/1
  Constant22/1 -> Product18/1, Product36/1
  Constant1/1 -> Math Function18/1
  Product1/1 -> Add10/3  "(delta6+z3)*sqrt(3)/2"
  Add15/1 -> Product74/1
  Add10/1 -> Math Function9/1  "XhPhi"
  Math Function7/1 -> Add3/3  "ZhPhi_2"
  rx/1 -> Product43/1, Product8/2, Product72/2, Product15/2, Product41/2, Product16/1, Product21/2, Product11/2  "rx"
  Product30/1 -> Add11/2  "r*sin(wt)*sqrt(3)/4"
  Sqrt7/1 -> Product4/1  "sqrt(3)"
  Product19/1 -> Trigonometric Function2/1, Trigonometric Function1/1
  Constant8/1 -> Product9/1, Sqrt7/1, Product19/2
  Constant9/1 -> Math Function8/2
  Math Function18/1 -> Add15/1  "10_exp(-100Dhp/r)"
  Constant5/1 -> Product10/2, Product4/2, Product3/1, Product6/2  "2"
  Constant2/1 -> Product9/2
  In2/1 -> Product1/2, Add7/2, Product3/2  "Z3 + delta6"
  Product22/1 -> NhPhix/DhPhix/1, Out1/1  "nhPhix/dhPhix"
  Product24/1 -> Add7/3  "r*sin(wt)*sqrt(3)/2"
  Trigonometric Function3/1 -> Product11/1  "sin(wt)"
  Product8/1 -> Add11/5  "r*sqrt(3)/4"
  Product5/1 -> Trigonometric Function6/1, Trigonometric Function3/1, Product19/1  "ai+wt"
  Trigonometric Function6/1 -> Product43/2  "cos(wt)"
  In1/1 -> Product17/2, Product23/2, Product36/2  "z6x"
  Math Function2/1 -> Add3/1
  Product35/1 -> Product74/2
  Clock/1 -> Product5/1
  Trigonometric Function1/1 -> Product16/2  "sin(3wt)"
  Product72/1 -> Math Function18/2
  Product41/1 -> Product14/2, Product2/1  "r*cos(3wt)"
  Product43/1 -> Product12/2, Product7/1  "r*cos(wt)"
  Add3/1 -> Sqrt1/1  "DhPhix_2"

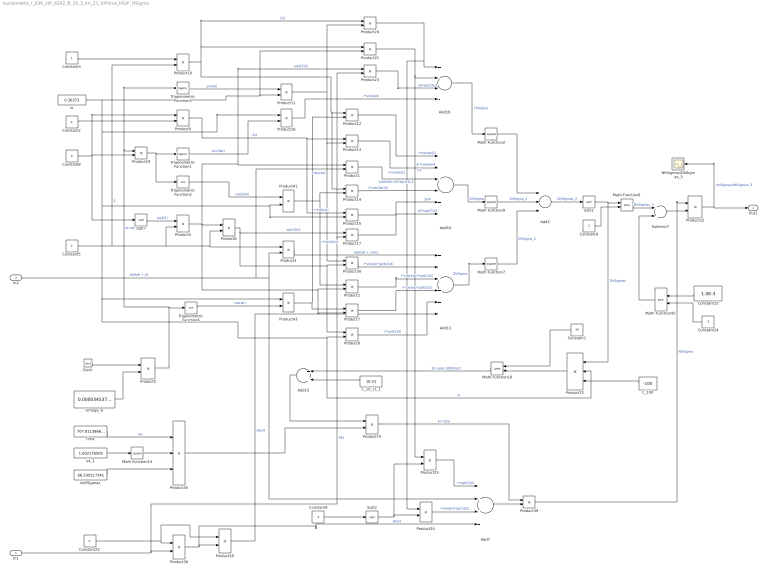
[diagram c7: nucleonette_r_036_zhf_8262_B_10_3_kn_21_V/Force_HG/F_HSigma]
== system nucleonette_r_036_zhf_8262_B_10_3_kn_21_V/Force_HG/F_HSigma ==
  In1 : Inport
  In2 : Inport  Port=2
  Add10 : Sum  Inputs=-++-++
  Add11 : Sum  Inputs=++++++
  Add15 : Sum
  Add19 : Sum  Inputs=+---
  Add3 : Sum  Inputs=+++
  Add7 : Sum  Inputs=++++
  C_100 : Constant  Value=-100
  C_10_11_1 : Constant  Value=1E-21
  Clock : Clock
  Constant1 : Constant  Value=10
  Constant15 : Constant  Value=1.0E-3
  Constant2 : Constant  Value=4
  Constant22 : Constant  Value=2
  Constant{4,8..9,24} (4 alike) : Constant  Value=3
  Constant3 : Constant
  Constant5 : Constant  Value=2
  Math Function{2,7,9,13} (4 alike) : Math  Operator=square
  Math Function18 : Math  Operator=pow
  Math Function45 : Math  Operator=pow
  Math Function8 : Math  Operator=pow
  NhSigmax/DhSigmax_3 : Scope
  Omega_w : Constant  Value=0.00003453723537
  Product{1,12..17,20..21,23..25,41,43,74} (15 alike) : Product  Inputs=**
  Product{4,6,9..10,22} (5 alike) : Product  Inputs=*/
  Product{2,5,7..8,11,19,30,39} (8 alike) : Product
  Product18 : Product  Inputs=/*
  Product3 : Product  Inputs=/*
  Product35 : Product  Inputs=/**
  Product36 : Product  Inputs=/*
  Product72 : Product  Inputs=*/*
  Sqrt1 : Sqrt
  Sqrt2 : Sqrt
  Sqrt7 : Sqrt
  Subtract7 : Sum
  Trigonometric Function1 : Trigonometry
  Trigonometric Function2 : Trigonometry  Operator=cos
  Trigonometric Function3 : Trigonometry
  Trigonometric Function6 : Trigonometry  Operator=cos
  ex_1 : Constant  Value=1.602176565
  keHSigmax : Constant  Value=66.535517341
  mHx : Constant  Value=707.811386658
  rx : Constant  Value=0.36373
  Out1 : Outport
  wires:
  Omega_w/1 -> Product5/2
  Subtract7/1 -> Product22/2
  Math Function8/1 -> Subtract7/1  "DhSigmax_3"
  Product22/1 -> NhSigmax/DhSigmax_3/1, Out1/1  "nhSigmax/dhSigmax_3"
  keHSigmax/1 -> Product35/3
  Trigonometric Function6/1 -> Product43/2  "cos(wt)"
  Add11/1 -> Math Function7/1  "ZhSigma"
  Product43/1 -> Product12/2, Product7/1  "r*cos(wt)"
  Product41/1 -> Product14/2, Product2/1  "r*cos(3wt)"
  Product11/1 -> Product13/2, Product30/1, Product20/2  "r*sin(wt)"
  Math Function13/1 -> Product35/2
  Math Function18/1 -> Add15/1  "10_exp(-100Dhs/r)"
  Trigonometric Function2/1 -> Product41/1  "cos(3wt)"
  Math Function9/1 -> Add3/2  "XhSigma_2"
  Constant8/1 -> Product9/1, Sqrt7/1, Product19/2
  Product39/1 -> Product22/1  "NhSigma"
  ex_1/1 -> Math Function13/1
  Product74/1 -> Product39/1  "kn_Dha"
  Trigonometric Function1/1 -> Product16/2  "sin(3wt)"
  Add3/1 -> Sqrt1/1  "DhSigmax_2"
  Math Function7/1 -> Add3/3  "ZhSigma_2"
  Constant22/1 -> Product18/1, Product36/1
  Math Function2/1 -> Add3/1
  rx/1 -> Product43/1, Product8/2, Product72/2, Product15/2, Product41/2, Product16/1, Product21/2, Product11/2  "rx"
  Clock/1 -> Product5/1
  Add10/1 -> Math Function9/1  "XhSigma"
  Product72/1 -> Math Function18/2
  Trigonometric Function3/1 -> Product11/1  "sin(wt)"
  Product19/1 -> Trigonometric Function2/1, Trigonometric Function1/1
  Constant5/1 -> Product10/2, Product4/2, Product3/1, Product6/2  "2"
  In2/1 -> Product1/2, Add7/2, Product3/2  "delta6 + z3"
  Product35/1 -> Product74/2
  C_10_11_1/1 -> Add15/2
  mHx/1 -> Product35/1  "mx"
  Add15/1 -> Product74/1
  Sqrt1/1 -> Math Function8/1, Product72/1  "DhSigmax"
  Sqrt7/1 -> Product4/1  "sqrt(3)"
  Constant9/1 -> Math Function8/2
  Add19/1 -> Math Function2/1  "YhSigma"
  Product30/1 -> Add11/2  "r*sin(wt)*sqrt(3)/4"
  Product5/1 -> Trigonometric Function6/1, Trigonometric Function3/1, Product19/1  "ai+wt"
  In1/1 -> Product17/2, Product23/2, Product36/2  "z6x"
  Add7/1 -> Product39/2
  C_100/1 -> Product72/3
  Constant1/1 -> Math Function18/1
  Constant15/1 -> Math Function45/1
  Constant24/1 -> Math Function45/2
  Math Function45/1 -> Subtract7/2
  Product3/1 -> Add11/1  "(delta6 + z3)/2"
  Product4/1 -> Product7/2, Product2/2, Product6/1, Product23/1, Product1/1  "sqrt(3)/2"
  Product6/1 -> Product17/1, Product8/1, Product30/2  "sqrt(3)/4"
  Product2/1 -> Add11/3  "r*cos(3wt)*sqrt(3)/2"
  Product7/1 -> Add11/4  "r*cos(wt)*sqrt(3)/2"
  Product8/1 -> Add11/5  "r*sqrt(3)/4"
  Constant2/1 -> Product9/2
  Constant3/1 -> Product10/1
  Product10/1 -> Product14/1, Product12/1, Product20/1, Product21/1  "1/2"
  Product12/1 -> Add10/1  "r*cos(wt)/2"
  Product9/1 -> Product15/1, Product13/1  "3/4"
  Product13/1 -> Add10/2  "3r*sin(wt)/4"
  Product1/1 -> Add10/3  "(delta6+z3)*sqrt(3)/2"
  Product14/1 -> Add10/4  "r*cos(3wt)/2"
  Product15/1 -> Add10/5  "3r/4"
  Product17/1 -> Add10/6  "z6*sqrt(3)/4"
  Product20/1 -> Add19/1, Product24/1  "r*sin(wt)/2"
  Product16/1 -> Add19/4  "r*sin(3wt)"
  Product21/1 -> Add19/2, Product25/1  "r/2"
  Product23/1 -> Add19/3  "z6*sqrt(3)/2"
  Product36/1 -> Add7/4, Product18/2  "z6x/2"
  Product18/1 -> Add11/6  "z6x/4"
  Product24/1 -> Add7/3  "r*sin(wt)*sqrt(3)/2"
  Sqrt2/1 -> Product25/2, Product24/2
  Constant4/1 -> Sqrt2/1
  Product25/1 -> Add7/1  "r*sqrt(3)/2"

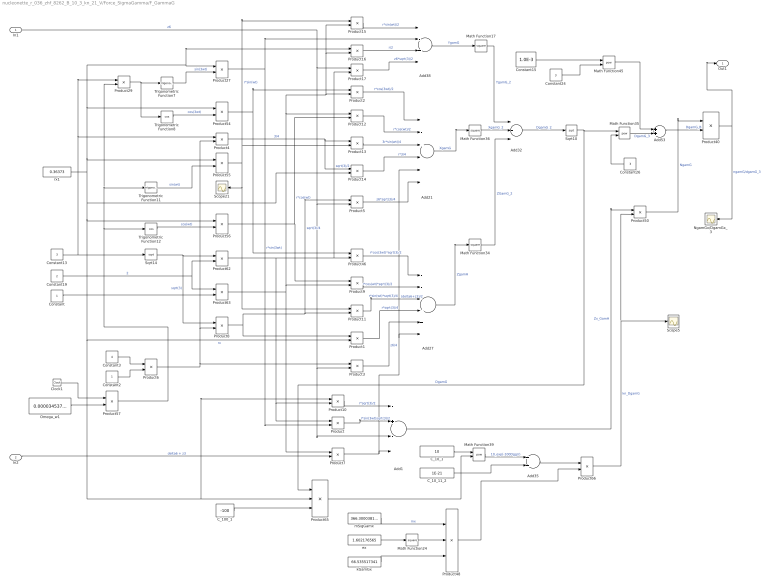
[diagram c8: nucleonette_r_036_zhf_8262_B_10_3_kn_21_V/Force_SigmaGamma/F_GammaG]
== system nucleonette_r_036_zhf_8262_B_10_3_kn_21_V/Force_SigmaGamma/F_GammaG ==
  In1 : Inport
  In2 : Inport  Port=2
  Add1 : Sum  Inputs=-+--
  Add21 : Sum  Inputs=--+---
  Add27 : Sum  Inputs=---+++
  Add32 : Sum  Inputs=+++
  Add35 : Sum
  Add38 : Sum  Inputs=+-++
  Add53 : Sum
  C_100_1 : Constant  Value=-100
  C_10_1 : Constant  Value=10
  C_10_11_2 : Constant  Value=1E-21
  Clock1 : Clock
  Constant : Constant
  Constant13 : Constant  Value=3
  Constant15 : Constant  Value=1.0E-3
  Constant19 : Constant  Value=2
  Constant2 : Constant
  Constant24 : Constant  Value=3
  Constant26 : Constant  Value=3
  Constant3 : Constant  Value=4
  Math Function{17,24,34,36} (4 alike) : Math  Operator=square
  Math Function35 : Math  Operator=pow
  Math Function39 : Math  Operator=pow
  Math Function45 : Math  Operator=pow
  NgamGx/DgamGx_3 : Scope
  Omega_w1 : Constant  Value=0.00003453723537
  Product{,1..5,7..17,29,46,50,57} (21 alike) : Product
  Product{27,54..56,66} (5 alike) : Product  Inputs=**
  Product40 : Product  Inputs=*/
  Product48 : Product  Inputs=/**
  Product6 : Product  Inputs=/*
  Product62 : Product  Inputs=*/
  Product63 : Product  Inputs=/*
  Product65 : Product  Inputs=*/*
  Scope21 : Scope
  Scope5 : Scope
  Sqrt10 : Sqrt
  Sqrt14 : Sqrt
  Trigonometric Function11 : Trigonometry
  Trigonometric Function12 : Trigonometry  Operator=cos
  Trigonometric Function7 : Trigonometry
  Trigonometric Function8 : Trigonometry  Operator=cos
  ex : Constant  Value=1.602176565
  kGamGx : Constant  Value=66.535517341
  mSigGamx : Constant  Value=366.300038182
  rx1 : Constant  Value=0.36373
  Out1 : Outport
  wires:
  Sqrt14/1 -> Product62/1, Product8/1  "sqrt(3)"
  Constant/1 -> Product63/2
  Constant2/1 -> Product6/2
  C_10_1/1 -> Math Function39/1
  Product50/1 -> Product40/1  "NgamG"
  Product27/1 -> Add38/2, Product/2  "r*sin(3wt)"
  ex/1 -> Math Function24/1
  rx1/1 -> Product16/1, Product27/1, Product54/1, Product55/1, Product14/2, Product1/2, Product65/2, Product10/1, Product56/1  "rx"
  kGamGx/1 -> Product48/3
  Constant15/1 -> Math Function45/1
  Constant24/1 -> Math Function45/2
  Trigonometric Function11/1 -> Product55/2  "sin(wt)"
  Product40/1 -> NgamGx/DgamGx_3/1, Out1/1  "ngamG/dgamG_3"
  Sqrt10/1 -> Product65/1, Math Function35/1  "DgamG"
  Product3/1 -> Add27/5  "z6/4"
  In1/1 -> Add1/3, Product3/2, Product5/2, Product17/1  "z6"
  Product17/1 -> Add38/4  "z6*sqrt(3)/2"
  Constant19/1 -> Product63/1, Product62/2  "2"
  Product15/1 -> Add38/1  "r*sin(wt)/2"
  Product16/1 -> Add38/3  "r/2"
  Math Function35/1 -> Add53/2  "DgamG_3"
  Trigonometric Function12/1 -> Product56/2  "cos(wt)"
  Product7/1 -> Add21/5, Add27/6, Add1/4  "(delta6+z3)/2"
  Trigonometric Function7/1 -> Product27/2  "sin(3wt)"
  In2/1 -> Product7/2  "delta6 + z3"
  Trigonometric Function8/1 -> Product54/2  "cos(3wt)"
  Constant13/1 -> Product4/1, Product29/1, Sqrt14/1
  Product14/1 -> Add21/4  "r*3/4"
  Product12/1 -> Add21/2  "r*cos(wt)/2"
  Math Function39/1 -> Add35/1  "10_exp(-100Dgg/r)"
  Product66/1 -> Scope5/1, Product50/2  "kn_DgamG"
  Product54/1 -> Product2/1, Product46/1
  Product5/1 -> Add21/6  "z6*sqrt(3)/4"
  Product10/1 -> Add1/1  "r*sqrt(3)/2"
  Math Function17/1 -> Add32/1  "YgamG_2"
  Omega_w1/1 -> Product57/2
  Product13/1 -> Add21/3  "3r*sin(wt)/4"
  Product4/1 -> Product13/1, Product14/1  "3/4"
  Add35/1 -> Product66/1
  Product2/1 -> Add21/1  "r*cos(3wt)/2"
  Product63/1 -> Product12/1, Product2/2, Product15/2, Product16/2, Product9/2, Product7/1
  Product65/1 -> Math Function39/2
  Constant26/1 -> Math Function35/2
  Math Function36/1 -> Add32/2  "XgamG_2"
  Product48/1 -> Product66/2
  Math Function24/1 -> Product48/2
  Product55/1 -> Product15/1, Product13/2, Scope21/1, Product11/1  "r*sin(wt)"
  mSigGamx/1 -> Product48/1  "mx"
  Math Function34/1 -> Add32/3  "ZGamG_2"
  Product56/1 -> Product12/2, Product9/1  "r*cos(wt)"
  Product11/1 -> Add27/3  "r*sin(wt)*sqrt(3)/4"
  Add38/1 -> Math Function17/1  "YgamG"
  Product1/1 -> Add27/4  "r*sqrt(3)/4"
  Product6/1 -> Product4/2, Product8/2, Product3/1
  Constant3/1 -> Product6/1
  Product8/1 -> Product11/2, Product5/1, Product1/1  "sqrt(3)/4"
  Add27/1 -> Math Function34/1  "ZgamH"
  Add53/1 -> Product40/2  "DgamG_B"
  C_100_1/1 -> Product65/3
  Add21/1 -> Math Function36/1  "XgamG"
  C_10_11_2/1 -> Add35/2
  Clock1/1 -> Product57/1
  Product57/1 -> Trigonometric Function12/1, Product29/2, Trigonometric Function11/1
  Product/1 -> Add1/2  "r*sin(3wt)sqrt(3)/2"
  Product9/1 -> Add27/2  "r*cos(wt)*sqrt(3)/2"
  Product62/1 -> Product/1, Product10/2, Product17/2, Product46/2  "sqrt(3)/2"
  Add32/1 -> Sqrt10/1  "DgamG_2"
  Product46/1 -> Add27/1  "r*cos(3wt)*sqrt(3)/2"
  Add1/1 -> Product50/1  "Zx_GamH"
  Math Function45/1 -> Add53/1
  Product29/1 -> Trigonometric Function8/1, Trigonometric Function7/1

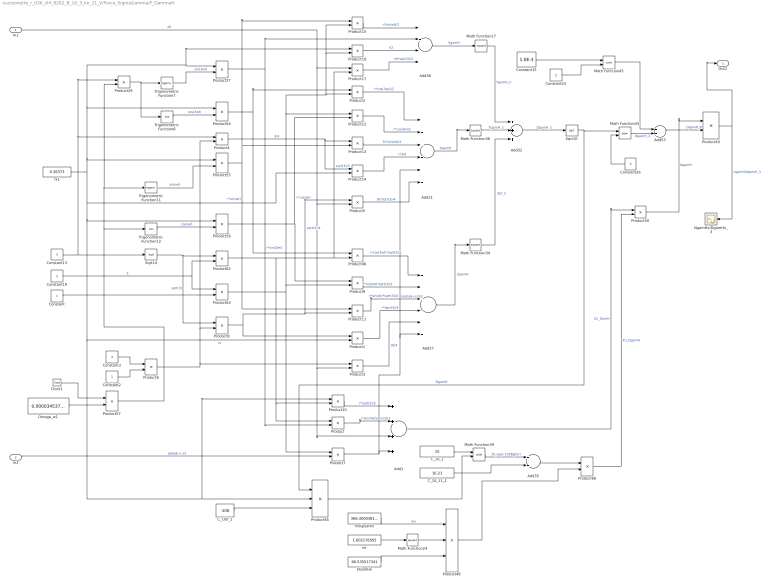
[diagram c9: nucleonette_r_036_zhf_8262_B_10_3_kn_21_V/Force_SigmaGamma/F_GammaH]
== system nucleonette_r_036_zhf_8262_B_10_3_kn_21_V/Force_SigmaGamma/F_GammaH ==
  In1 : Inport
  In2 : Inport  Port=2
  Add1 : Sum  Inputs=++++
  Add21 : Sum  Inputs=-+-+++
  Add27 : Sum  Inputs=-++---
  Add32 : Sum  Inputs=+++
  Add35 : Sum
  Add38 : Sum  Inputs=----
  Add53 : Sum
  C_100_1 : Constant  Value=-100
  C_10_1 : Constant  Value=10
  C_10_11_2 : Constant  Value=1E-21
  Clock1 : Clock
  Constant : Constant
  Constant13 : Constant  Value=3
  Constant15 : Constant  Value=1.0E-3
  Constant19 : Constant  Value=2
  Constant2 : Constant
  Constant24 : Constant  Value=3
  Constant26 : Constant  Value=3
  Constant3 : Constant  Value=4
  Math Function{17,24,34,36} (4 alike) : Math  Operator=square
  Math Function35 : Math  Operator=pow
  Math Function39 : Math  Operator=pow
  Math Function45 : Math  Operator=pow
  NgamHx/DgamHx_3 : Scope
  Omega_w1 : Constant  Value=0.00003453723537
  Product{,1..5,7..17,29,46,50,57} (21 alike) : Product
  Product{27,54..56,66} (5 alike) : Product  Inputs=**
  Product40 : Product  Inputs=*/
  Product48 : Product  Inputs=/**
  Product6 : Product  Inputs=/*
  Product62 : Product  Inputs=*/
  Product63 : Product  Inputs=/*
  Product65 : Product  Inputs=*/*
  Sqrt10 : Sqrt
  Sqrt14 : Sqrt
  Trigonometric Function11 : Trigonometry
  Trigonometric Function12 : Trigonometry  Operator=cos
  Trigonometric Function7 : Trigonometry
  Trigonometric Function8 : Trigonometry  Operator=cos
  ex : Constant  Value=1.602176565
  kGamHx : Constant  Value=66.535517341
  mSigGamx : Constant  Value=366.300038182
  rx1 : Constant  Value=0.36373
  Out1 : Outport
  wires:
  Add1/1 -> Product50/1  "Zx_GamH"
  Math Function34/1 -> Add32/3  "Zbf_2"
  Product48/1 -> Product66/2
  Add38/1 -> Math Function17/1  "XgamH"
  Math Function24/1 -> Product48/2
  Trigonometric Function7/1 -> Product27/2  "sin(3wt)"
  Add35/1 -> Product66/1
  Constant/1 -> Product63/2
  Product54/1 -> Product2/1, Product46/1
  Product56/1 -> Product12/2, Product9/1  "r*cos(wt)"
  C_10_11_2/1 -> Add35/2
  Product62/1 -> Product/1, Product10/2, Product17/2, Product46/2  "sqrt(3)/2"
  Product40/1 -> NgamHx/DgamHx_3/1, Out1/1  "ngamH/dgamH_3"
  Constant19/1 -> Product63/1, Product62/2  "2"
  Add53/1 -> Product40/2  "DgamH_B"
  Sqrt14/1 -> Product62/1, Product8/1  "sqrt(3)"
  Sqrt10/1 -> Product65/1, Math Function35/1  "DgamH"
  Product63/1 -> Product12/1, Product2/2, Product15/2, Product16/2, Product9/2, Product7/1
  Add32/1 -> Sqrt10/1  "DgamH_2"
  In1/1 -> Add1/3, Product3/2, Product5/2, Product17/1  "z6"
  In2/1 -> Product7/2  "delta6 + z3"
  Product57/1 -> Trigonometric Function12/1, Product29/2, Trigonometric Function11/1
  C_10_1/1 -> Math Function39/1
  Math Function39/1 -> Add35/1  "10_exp(-100Dgh/r)"
  Math Function45/1 -> Add53/1
  mSigGamx/1 -> Product48/1  "mx"
  Omega_w1/1 -> Product57/2
  Product66/1 -> Product50/2  "kn_DgamH"
  Product55/1 -> Product15/1, Product13/2, Product11/1  "r*sin(wt)"
  Trigonometric Function8/1 -> Product54/2  "cos(3wt)"
  Trigonometric Function12/1 -> Product56/2  "cos(wt)"
  Trigonometric Function11/1 -> Product55/2  "sin(wt)"
  Math Function36/1 -> Add32/2  "XgamH_2"
  Constant24/1 -> Math Function45/2
  Constant15/1 -> Math Function45/1
  Add21/1 -> Math Function36/1  "XgamH"
  Product29/1 -> Trigonometric Function8/1, Trigonometric Function7/1
  C_100_1/1 -> Product65/3
  Clock1/1 -> Product57/1
  Add27/1 -> Math Function34/1  "ZgamH"
  Product5/1 -> Add21/6  "z6*sqrt(3)/4"
  rx1/1 -> Product16/1, Product27/1, Product54/1, Product55/1, Product14/2, Product1/2, Product65/2, Product10/1, Product56/1  "rx"
  kGamHx/1 -> Product48/3
  ex/1 -> Math Function24/1
  Math Function17/1 -> Add32/1  "YgamH_2"
  Product65/1 -> Math Function39/2
  Math Function35/1 -> Add53/2  "DgamH_3"
  Product46/1 -> Add27/1  "r*cos(3wt)*sqrt(3)/2"
  Product50/1 -> Product40/1  "NgamH"
  Product27/1 -> Add38/2, Product/2  "r*sin(3wt)"
  Constant26/1 -> Math Function35/2
  Product/1 -> Add1/2  "r*sin(3wt)sqrt(3)/2"
  Constant2/1 -> Product6/2
  Constant3/1 -> Product6/1
  Product6/1 -> Product4/2, Product8/2, Product3/1
  Product10/1 -> Add1/1  "r*sqrt(3)/2"
  Product3/1 -> Add27/5  "z6/4"
  Product9/1 -> Add27/2  "r*cos(wt)*sqrt(3)/2"
  Product8/1 -> Product11/2, Product5/1, Product1/1  "sqrt(3)/4"
  Product1/1 -> Add27/4  "r*sqrt(3)/4"
  Product11/1 -> Add27/3  "r*sin(wt)*sqrt(3)/4"
  Product2/1 -> Add21/1  "r*cos(3wt)/2"
  Product12/1 -> Add21/2  "r*cos(wt)/2"
  Constant13/1 -> Product4/1, Product29/1, Sqrt14/1
  Product4/1 -> Product13/1, Product14/1  "3/4"
  Product13/1 -> Add21/3  "3r*sin(wt)/4"
  Product14/1 -> Add21/4  "r*3/4"
  Product7/1 -> Add21/5, Add27/6, Add1/4  "(delta6+z3)/2"
  Product15/1 -> Add38/1  "r*sin(wt)/2"
  Product16/1 -> Add38/3  "r/2"
  Product17/1 -> Add38/4  "z6*sqrt(3)/2"
